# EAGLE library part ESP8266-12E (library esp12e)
ESP8266-12E Library for Eagle CAD The author not responsible for any damages or errors!. Created by Suhail jr.lt;/author>
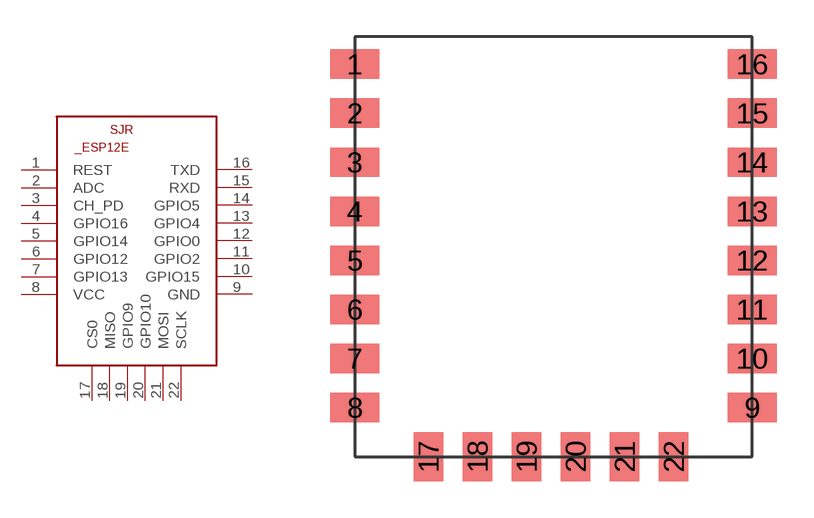
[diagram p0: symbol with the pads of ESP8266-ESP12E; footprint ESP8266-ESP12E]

Designator prefix SJR

## ESP8266-12EESP12E  [ESP8266-ESP12E]
1  REST
2  ADC
3  CH_PD
4  GPIO16
5  GPIO14
6  GPIO12
7  GPIO13
8  VCC
9  GND
10  GPIO15
11  GPIO2
12  GPIO0
13  GPIO4
14  GPIO5
15  RXD
16  TXD
17  CS0
18  MISO
19  GPIO9
20  GPIO10
21  MOSI
22  SCLK

## Footprint ESP8266-ESP12E (pad centres in mm)
ESP8266-12E Library for Eagle CAD The author not responsible for any damages or errors!. Created by Suhail jr.lt;/author>
smd 2 x 1.2: 1 -7.62,5.84; 2 -7.62,3.84; 3 -7.62,1.84; 4 -7.62,-0.16; 5 -7.62,-2.16; 6 -7.62,-4.16; 7 -7.62,-6.16; 8 -7.62,-8.16; 9 8.58,-8.16; 10 8.58,-6.16; 11 8.58,-4.16; 12 8.58,-2.16; 13 8.58,-0.16; 14 8.58,1.84; 15 8.58,3.84; 16 8.58,5.84
smd 1.2 x 2: 17 -4.62,-10.16; 18 -2.62,-10.16; 19 -0.62,-10.16; 20 1.38,-10.16; 21 3.38,-10.16; 22 5.38,-10.16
